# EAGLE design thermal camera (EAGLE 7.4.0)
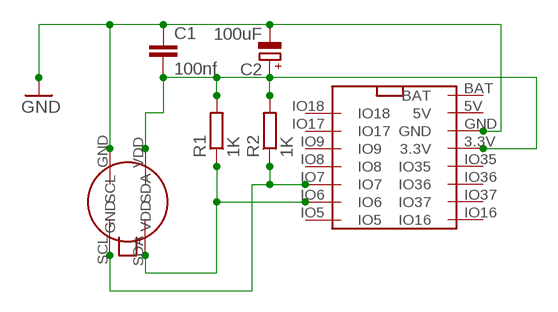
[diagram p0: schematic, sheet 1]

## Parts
C1  100nf  C-EUC0805  [C0805]
C2  100uF  CPOL-EUE2-5  [E2-5]
R1  1K  R-EU_R0805  [R0805]
R2  1K  R-EU_R0805  [R0805]
U$1  01SPACE-ESP32S3  [01SPACE-ESP32S3]
U$2  MLX90640  [MLX90640]

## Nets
GND: C1.1 C2.- U$1.GND U$2.GND
N$2: C1.2 C2.+ R1.2 R2.2 U$1.3.3V U$2.VDD
N$3: R1.1 U$1.IO6 U$2.SDA
N$4: R2.1 U$1.IO7 U$2.SCL
Unconnected: U$1.5V U$1.BAT U$1.IO5 U$1.IO8 U$1.IO9 U$1.IO16 U$1.IO17 U$1.IO18 U$1.IO35 U$1.IO36 U$1.IO37

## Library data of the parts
C1 = resistor:C-EU: CAPACITOR, European symbol
C2 = resistor:CPOL-EU: POLARIZED CAPACITOR, European symbol
R1 R2 = resistor:R-EU_: RESISTOR, European symbol
U$1 = perso:01SPACE-ESP32S3
U$2 = perso:MLX90640

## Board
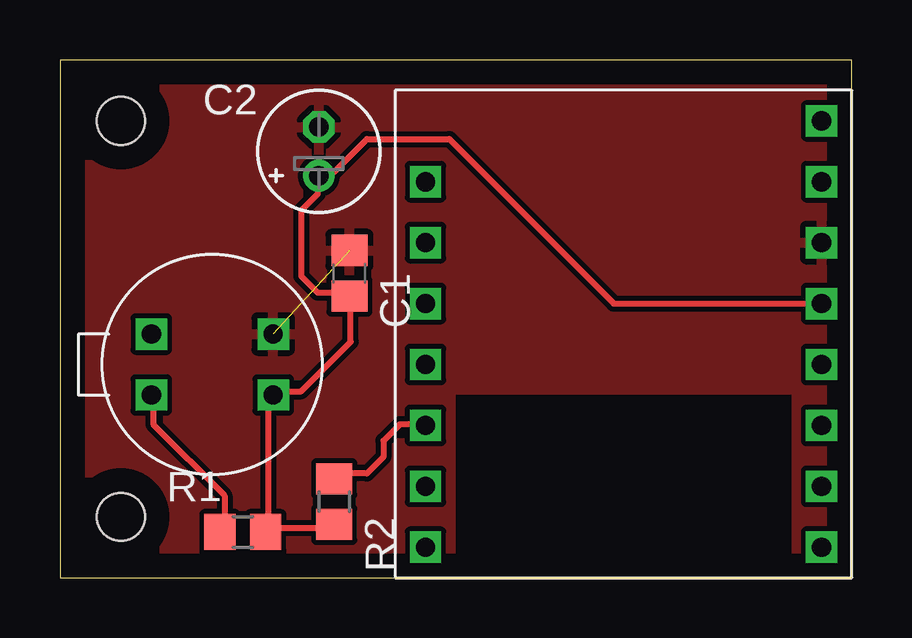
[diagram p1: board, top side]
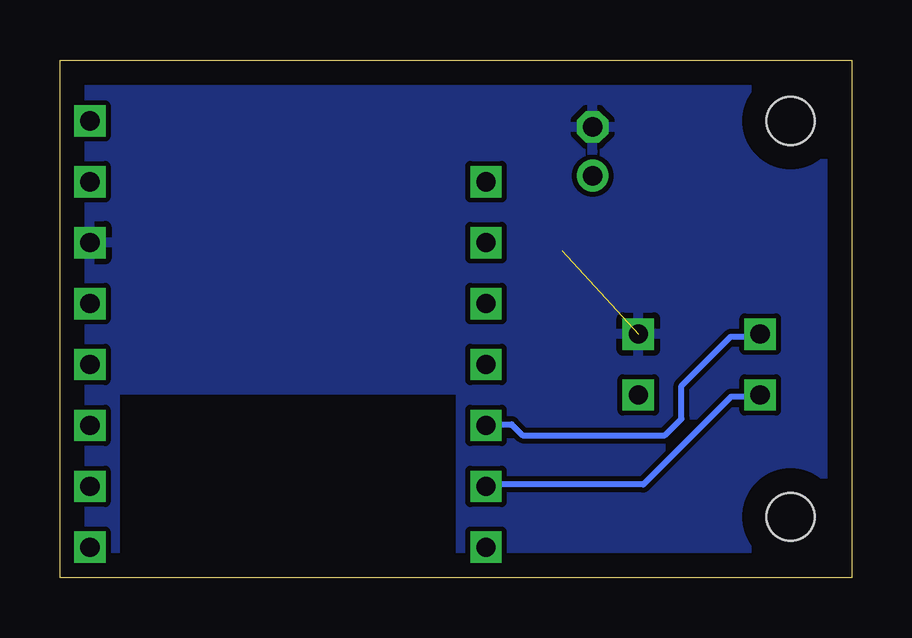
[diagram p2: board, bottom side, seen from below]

Size 33 x 21.59 mm. Coordinates in mm from the lower left corner, seen from the top.
Outline: 0,0 33,0 33,21.59 0,21.59 0,0
Copper layers (1*16): Top 0.035mm / dielectric 1.5mm / Bottom 0.035mm
Design rules "default": minimum track width 10mil, minimum drill 24mil, track to track 8mil, track to pad 8mil, pad to pad 8mil, via to via 8mil, smd to smd 8mil, copper to edge 40mil, drill to drill 8mil, minimum pad ring 10mil, minimum via ring 8mil, stop-mask expansion 4mil, vias tented up to drill 0mil, thermal gap 10mil
Holes 2 mm at 2.54,2.54 2.54,19.05
tRestrict: area 16.5,0 to 30.5,7.6
bRestrict: area 16.5,0 to 30.5,7.6

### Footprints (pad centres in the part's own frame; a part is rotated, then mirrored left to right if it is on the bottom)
C0805 = smd 1.3 x 1.5: 1 -0.95,0; 2 0.95,0
E2-5 = drill 0.813 pad 1.27: + -1.016,0 | drill 0.813 pad 1.27 octagon: - 1.016,0
R0805 = smd 1.3 x 1.5: 1 -0.95,0; 2 0.95,0
01SPACE-ESP32S3 = drill 0.8 square: 3.3V 5.08,0; 5V 5.08,5.08; BAT 5.08,7.62; GND 5.08,2.54; IO5 -11.43,-10.16; IO6 -11.43,-7.62; IO7 -11.43,-5.08; IO8 -11.43,-2.54; IO9 -11.43,0; IO16 5.08,-10.16; IO17 -11.43,2.54; IO18 -11.43,5.08; IO35 5.08,-2.54; IO36 5.08,-5.08; IO37 5.08,-7.62
MLX90640 = drill 0.8 square: GND 2.54,1.27; SCL -2.54,1.27; SDA -2.54,-1.27; VDD 2.54,-1.27

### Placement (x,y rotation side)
C1  12.06,12.7 270 top
C2  10.79,17.78 90 top
R1  7.62,1.91 0 top
R2  11.43,3.17 270 top
U$1  26.67,11.43 0 top
U$2  6.35,8.89 0 top

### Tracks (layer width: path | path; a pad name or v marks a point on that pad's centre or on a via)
GND  (1 unrouted)
  pour Top: 33.02,21.59 0,21.59 0,0 33.02,0
  pour Bottom: 33.02,21.59 0,21.59 0,0 33.02,0
N$2
  Top 0.254: 8.69,2.06 11.43,2.06 R2.2 | 8.69,2.06 8.69,7.54 U$2.VDD 8.91,7.77 10.06,7.77 12.12,9.83 12.12,11.66 C1.2 11.89,11.89 10.74,11.89 10.06,12.57 10.06,15.32 10.74,16 10.74,16.69 C2.+ 10.97,16.92 11.43,16.92 12.8,18.29 16.23,18.29 23.09,11.43 U$1.3.3V | 8.69,2.06 R1.2
N$3
  Top 0.254: R1.1 6.86,2.06 6.86,3.43 3.89,6.4 3.89,7.54 U$2.SDA
  Bottom 0.254: U$1.IO6 15.09,3.89 8.69,3.89 5.03,7.54 3.89,7.54 U$2.SDA
N$4
  Top 0.254: R2.1 11.43,4.34 12.8,4.34 13.49,5.03 13.49,5.71 14.17,6.4 15.09,6.4 U$1.IO7
  Bottom 0.254: U$2.SCL 3.89,10.06 5.03,10.06 7.09,8 7.09,6.63 7.77,5.94 13.72,5.94 14.17,6.4 15.09,6.4 U$1.IO7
